ORGANIZATION_BLOCK "Organizzazione Blocchi"
TITLE = "Main Program Sweep (Cycle)"
AUTHOR : MassimoZ
VERSION : 0.1


VAR_TEMP
  OB1_EV_CLASS : BYTE ;	//Bits 0-3 = 1 (Coming event), Bits 4-7 = 1 (Event class 1)
  OB1_SCAN_1 : BYTE ;	//1 (Cold restart scan 1 of OB 1), 3 (Scan 2-n of OB 1)
  OB1_PRIORITY : BYTE ;	//1 (Priority of 1 is lowest)
  OB1_OB_NUMBR : BYTE ;	//1 (Organization block 1, OB1)
  OB1_RESERVED_1 : BYTE ;	//Reserved for system
  OB1_RESERVED_2 : BYTE ;	//Reserved for system
  OB1_PREV_CYCLE : INT ;	//Cycle time of previous OB1 scan (milliseconds)
  OB1_MIN_CYCLE : INT ;	//Minimum cycle time of OB1 (milliseconds)
  OB1_MAX_CYCLE : INT ;	//Maximum cycle time of OB1 (milliseconds)
  OB1_DATE_TIME : DATE_AND_TIME ;	//Date and time OB1 started
END_VAR
BEGIN
NETWORK
TITLE =Lettura Data / Ora

      L     LD    12;
      T     DB100.DBD    2;
NETWORK
TITLE =Gestione Posizioni

      UC    "Gest Posizioni";

NETWORK
TITLE =Gestione Consensi

      UC    "Gest Consensi";

NETWORK
TITLE =Gestione Pulsantiera

      UC    "Gest Pulsantiera";

NETWORK
TITLE =Gestione Manuali

      UC    "Gest Manuali";

NETWORK
TITLE =Gestione Semi Automatico

      UC    "Gest Semi Automatico";

NETWORK
TITLE =Gestione Automatico

      UC    "Gest Automatico";

NETWORK
TITLE =Gestione Avvisi / Allarmi

      UC    "Gest Avvisi/Allarmi";

NETWORK
TITLE =Gestione Interfaccie

      UC    "Gest Interfaccie";

NETWORK
TITLE =Gestione Reset

      UC    "Gest Reset";

NETWORK
TITLE =Gestione Output

      UC    "Gest Output";

NETWORK
TITLE =Gest Trasmissione Dati Rete Supervisore Crimpatura/Spazzolatura
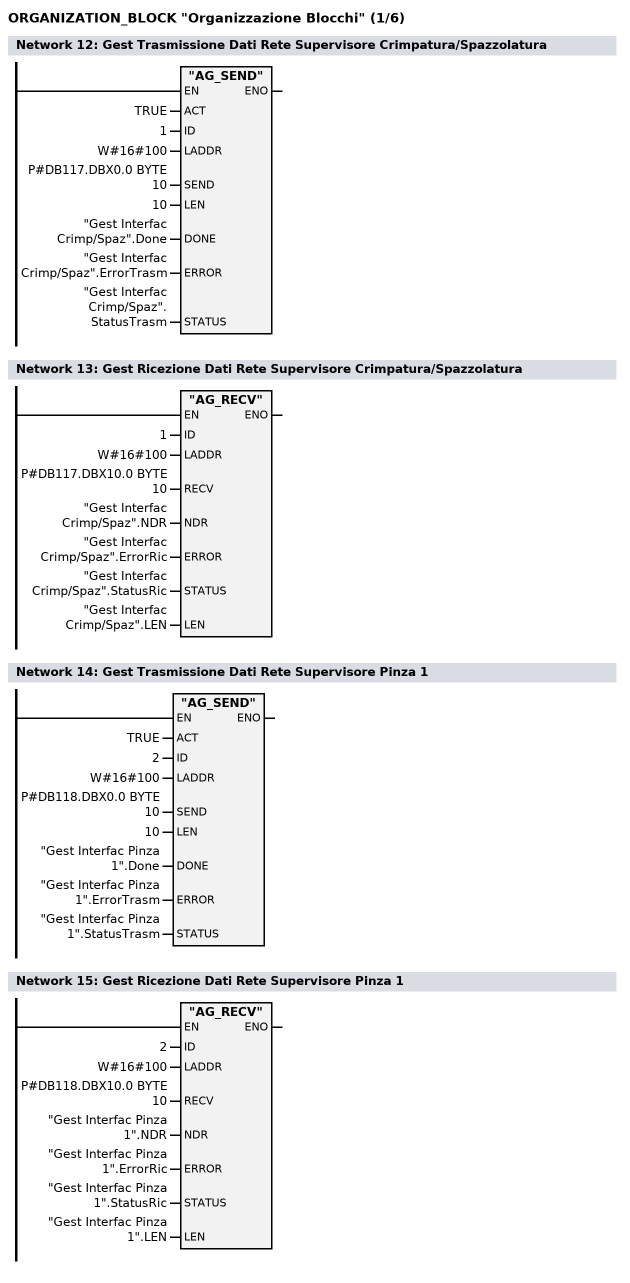
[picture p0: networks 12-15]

      CALL "AG_SEND" (
           ACT                      := TRUE,
           ID                       := 1,
           LADDR                    := W#16#100,
           SEND                     := P#DB117.DBX0.0 BYTE 10,
           LEN                      := 10,
           DONE                     := "Gest Interfac Crimp/Spaz".Done,
           ERROR                    := "Gest Interfac Crimp/Spaz".ErrorTrasm,
           STATUS                   := "Gest Interfac Crimp/Spaz".StatusTrasm);

NETWORK
TITLE =Gest Ricezione Dati Rete Supervisore Crimpatura/Spazzolatura

      CALL "AG_RECV" (
           ID                       := 1,
           LADDR                    := W#16#100,
           RECV                     := P#DB117.DBX10.0 BYTE 10,
           NDR                      := "Gest Interfac Crimp/Spaz".NDR,
           ERROR                    := "Gest Interfac Crimp/Spaz".ErrorRic,
           STATUS                   := "Gest Interfac Crimp/Spaz".StatusRic,
           LEN                      := "Gest Interfac Crimp/Spaz".LEN);

NETWORK
TITLE =Gest Trasmissione Dati Rete Supervisore Pinza 1

      CALL "AG_SEND" (
           ACT                      := TRUE,
           ID                       := 2,
           LADDR                    := W#16#100,
           SEND                     := P#DB118.DBX0.0 BYTE 10,
           LEN                      := 10,
           DONE                     := "Gest Interfac Pinza 1".Done,
           ERROR                    := "Gest Interfac Pinza 1".ErrorTrasm,
           STATUS                   := "Gest Interfac Pinza 1".StatusTrasm);

NETWORK
TITLE =Gest Ricezione Dati Rete Supervisore Pinza 1

      CALL "AG_RECV" (
           ID                       := 2,
           LADDR                    := W#16#100,
           RECV                     := P#DB118.DBX10.0 BYTE 10,
           NDR                      := "Gest Interfac Pinza 1".NDR,
           ERROR                    := "Gest Interfac Pinza 1".ErrorRic,
           STATUS                   := "Gest Interfac Pinza 1".StatusRic,
           LEN                      := "Gest Interfac Pinza 1".LEN);

NETWORK
TITLE =Gest Trasmissione Dati Rete Supervisore Pinza 2
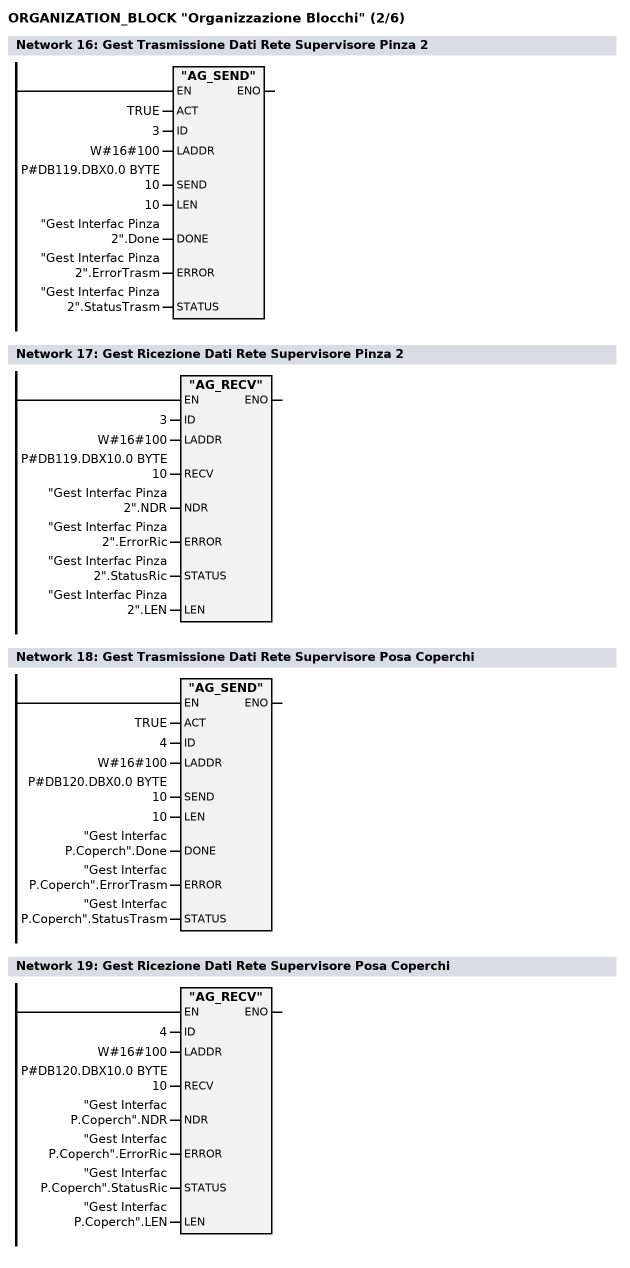
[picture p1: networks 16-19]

      CALL "AG_SEND" (
           ACT                      := TRUE,
           ID                       := 3,
           LADDR                    := W#16#100,
           SEND                     := P#DB119.DBX0.0 BYTE 10,
           LEN                      := 10,
           DONE                     := "Gest Interfac Pinza 2".Done,
           ERROR                    := "Gest Interfac Pinza 2".ErrorTrasm,
           STATUS                   := "Gest Interfac Pinza 2".StatusTrasm);

NETWORK
TITLE =Gest Ricezione Dati Rete Supervisore Pinza 2

      CALL "AG_RECV" (
           ID                       := 3,
           LADDR                    := W#16#100,
           RECV                     := P#DB119.DBX10.0 BYTE 10,
           NDR                      := "Gest Interfac Pinza 2".NDR,
           ERROR                    := "Gest Interfac Pinza 2".ErrorRic,
           STATUS                   := "Gest Interfac Pinza 2".StatusRic,
           LEN                      := "Gest Interfac Pinza 2".LEN);

NETWORK
TITLE =Gest Trasmissione Dati Rete Supervisore Posa Coperchi

      CALL "AG_SEND" (
           ACT                      := TRUE,
           ID                       := 4,
           LADDR                    := W#16#100,
           SEND                     := P#DB120.DBX0.0 BYTE 10,
           LEN                      := 10,
           DONE                     := "Gest Interfac P.Coperch".Done,
           ERROR                    := "Gest Interfac P.Coperch".ErrorTrasm,
           STATUS                   := "Gest Interfac P.Coperch".StatusTrasm);

NETWORK
TITLE =Gest Ricezione Dati Rete Supervisore Posa Coperchi

      CALL "AG_RECV" (
           ID                       := 4,
           LADDR                    := W#16#100,
           RECV                     := P#DB120.DBX10.0 BYTE 10,
           NDR                      := "Gest Interfac P.Coperch".NDR,
           ERROR                    := "Gest Interfac P.Coperch".ErrorRic,
           STATUS                   := "Gest Interfac P.Coperch".StatusRic,
           LEN                      := "Gest Interfac P.Coperch".LEN);

NETWORK
TITLE =Gest Trasmissione Dati Rete Supervisore Termo 1
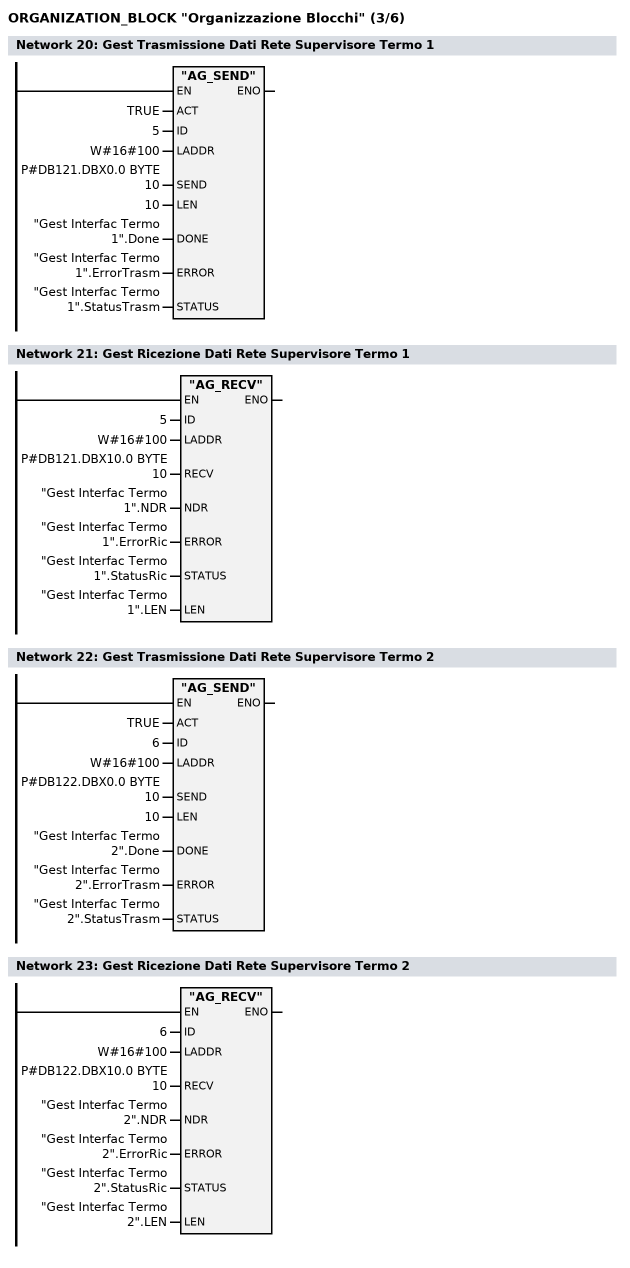
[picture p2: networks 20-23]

      CALL "AG_SEND" (
           ACT                      := TRUE,
           ID                       := 5,
           LADDR                    := W#16#100,
           SEND                     := P#DB121.DBX0.0 BYTE 10,
           LEN                      := 10,
           DONE                     := "Gest Interfac Termo 1".Done,
           ERROR                    := "Gest Interfac Termo 1".ErrorTrasm,
           STATUS                   := "Gest Interfac Termo 1".StatusTrasm);

NETWORK
TITLE =Gest Ricezione Dati Rete Supervisore Termo 1

      CALL "AG_RECV" (
           ID                       := 5,
           LADDR                    := W#16#100,
           RECV                     := P#DB121.DBX10.0 BYTE 10,
           NDR                      := "Gest Interfac Termo 1".NDR,
           ERROR                    := "Gest Interfac Termo 1".ErrorRic,
           STATUS                   := "Gest Interfac Termo 1".StatusRic,
           LEN                      := "Gest Interfac Termo 1".LEN);

NETWORK
TITLE =Gest Trasmissione Dati Rete Supervisore Termo 2

      CALL "AG_SEND" (
           ACT                      := TRUE,
           ID                       := 6,
           LADDR                    := W#16#100,
           SEND                     := P#DB122.DBX0.0 BYTE 10,
           LEN                      := 10,
           DONE                     := "Gest Interfac Termo 2".Done,
           ERROR                    := "Gest Interfac Termo 2".ErrorTrasm,
           STATUS                   := "Gest Interfac Termo 2".StatusTrasm);

NETWORK
TITLE =Gest Ricezione Dati Rete Supervisore Termo 2

      CALL "AG_RECV" (
           ID                       := 6,
           LADDR                    := W#16#100,
           RECV                     := P#DB122.DBX10.0 BYTE 10,
           NDR                      := "Gest Interfac Termo 2".NDR,
           ERROR                    := "Gest Interfac Termo 2".ErrorRic,
           STATUS                   := "Gest Interfac Termo 2".StatusRic,
           LEN                      := "Gest Interfac Termo 2".LEN);

NETWORK
TITLE =Gest Trasmissione Dati Rete Supervisore Pneumo 1
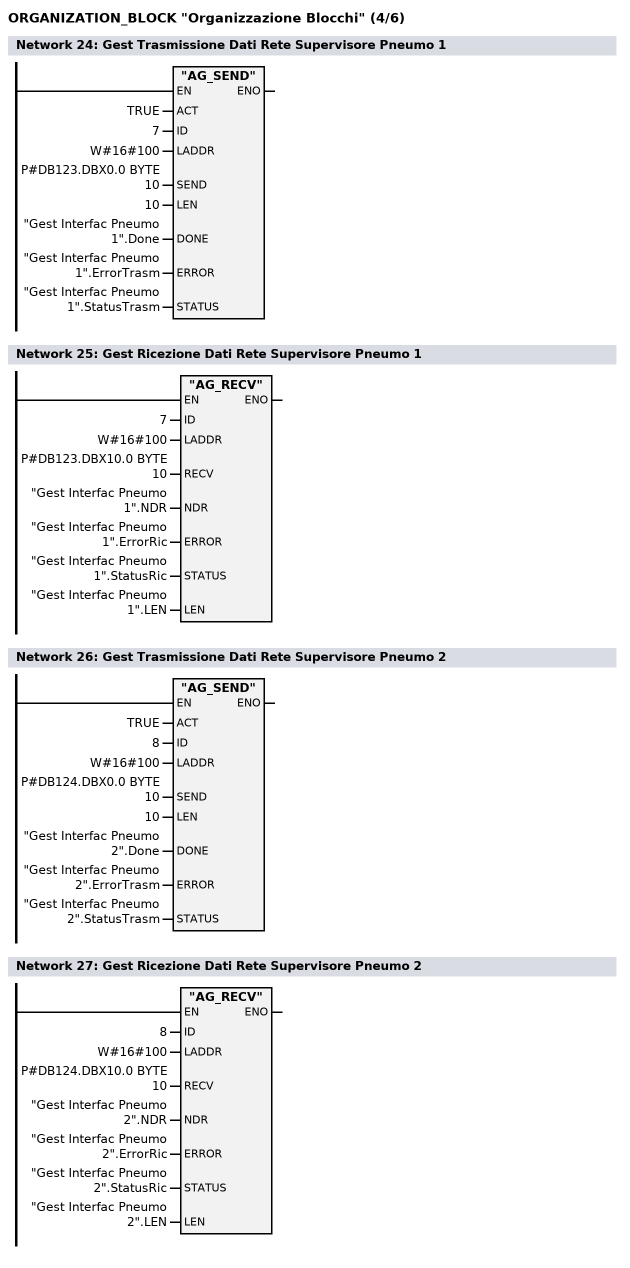
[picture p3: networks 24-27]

      CALL "AG_SEND" (
           ACT                      := TRUE,
           ID                       := 7,
           LADDR                    := W#16#100,
           SEND                     := P#DB123.DBX0.0 BYTE 10,
           LEN                      := 10,
           DONE                     := "Gest Interfac Pneumo 1".Done,
           ERROR                    := "Gest Interfac Pneumo 1".ErrorTrasm,
           STATUS                   := "Gest Interfac Pneumo 1".StatusTrasm);

NETWORK
TITLE =Gest Ricezione Dati Rete Supervisore Pneumo 1

      CALL "AG_RECV" (
           ID                       := 7,
           LADDR                    := W#16#100,
           RECV                     := P#DB123.DBX10.0 BYTE 10,
           NDR                      := "Gest Interfac Pneumo 1".NDR,
           ERROR                    := "Gest Interfac Pneumo 1".ErrorRic,
           STATUS                   := "Gest Interfac Pneumo 1".StatusRic,
           LEN                      := "Gest Interfac Pneumo 1".LEN);

NETWORK
TITLE =Gest Trasmissione Dati Rete Supervisore Pneumo 2

      CALL "AG_SEND" (
           ACT                      := TRUE,
           ID                       := 8,
           LADDR                    := W#16#100,
           SEND                     := P#DB124.DBX0.0 BYTE 10,
           LEN                      := 10,
           DONE                     := "Gest Interfac Pneumo 2".Done,
           ERROR                    := "Gest Interfac Pneumo 2".ErrorTrasm,
           STATUS                   := "Gest Interfac Pneumo 2".StatusTrasm);

NETWORK
TITLE =Gest Ricezione Dati Rete Supervisore Pneumo 2

      CALL "AG_RECV" (
           ID                       := 8,
           LADDR                    := W#16#100,
           RECV                     := P#DB124.DBX10.0 BYTE 10,
           NDR                      := "Gest Interfac Pneumo 2".NDR,
           ERROR                    := "Gest Interfac Pneumo 2".ErrorRic,
           STATUS                   := "Gest Interfac Pneumo 2".StatusRic,
           LEN                      := "Gest Interfac Pneumo 2".LEN);

NETWORK
TITLE =
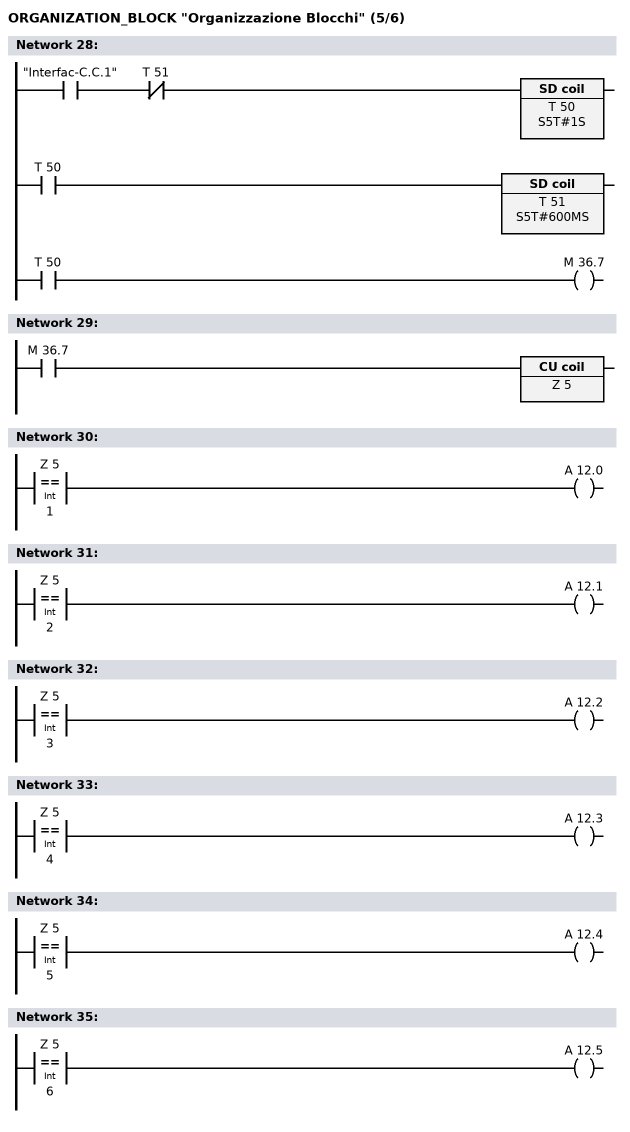
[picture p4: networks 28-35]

      U     "Interfac-C.C.1";
      UN    T     51;
      L     S5T#1S;
      SE    T     50;
      U     T     50;
      L     S5T#600MS;
      SE    T     51;
      U     T     50;
      =     M     36.7;
NETWORK
TITLE =

      U     M     36.7;
      ZV    Z      5;
NETWORK
TITLE =

      L     Z      5;
      L     1;
      ==I   ;
      =     A     12.0;
NETWORK
TITLE =

      L     Z      5;
      L     2;
      ==I   ;
      =     A     12.1;
NETWORK
TITLE =

      L     Z      5;
      L     3;
      ==I   ;
      =     A     12.2;
NETWORK
TITLE =

      L     Z      5;
      L     4;
      ==I   ;
      =     A     12.3;
NETWORK
TITLE =

      L     Z      5;
      L     5;
      ==I   ;
      =     A     12.4;
NETWORK
TITLE =

      L     Z      5;
      L     6;
      ==I   ;
      =     A     12.5;
NETWORK
TITLE =Contatore al preset
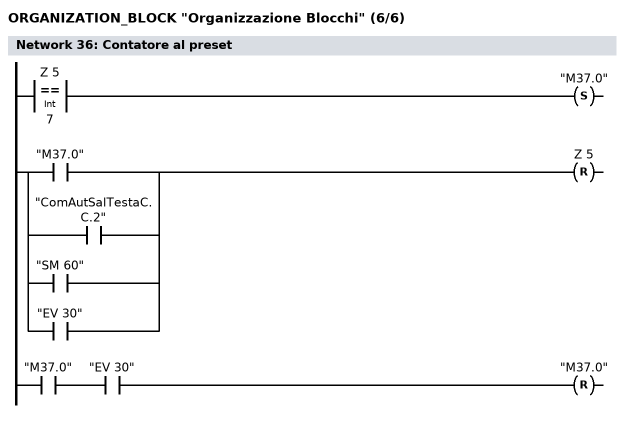
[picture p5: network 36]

      L     Z      5;
      L     7;
      ==I   ;
      S     "M37.0";
      U     "M37.0";
      O     "ComAutSalTestaC.C.2";
      O     "SM 60";
      O     "EV 30";
      R     Z      5;
      U     "M37.0";
      U     "EV 30";
      R     "M37.0";
NETWORK
TITLE =

      UC    FC   101;

      CALL FC   103 ;


NETWORK
TITLE =

      UC    FC   110;

NETWORK
TITLE =
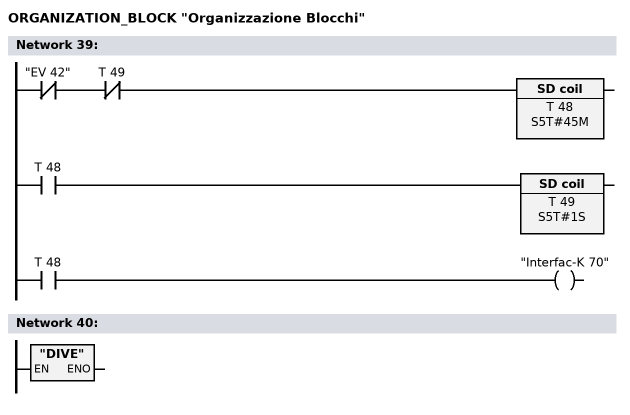
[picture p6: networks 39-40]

      UN    "EV 42";
      UN    T     49;
      L     S5T#45M;
      SE    T     48;
      U     T     48;
      L     S5T#1S;
      SE    T     49;
      U     T     48;
      =     "Interfac-K 70";
NETWORK
TITLE =

      CALL "DIVE" ;

NETWORK
TITLE =



END_ORGANIZATION_BLOCK

